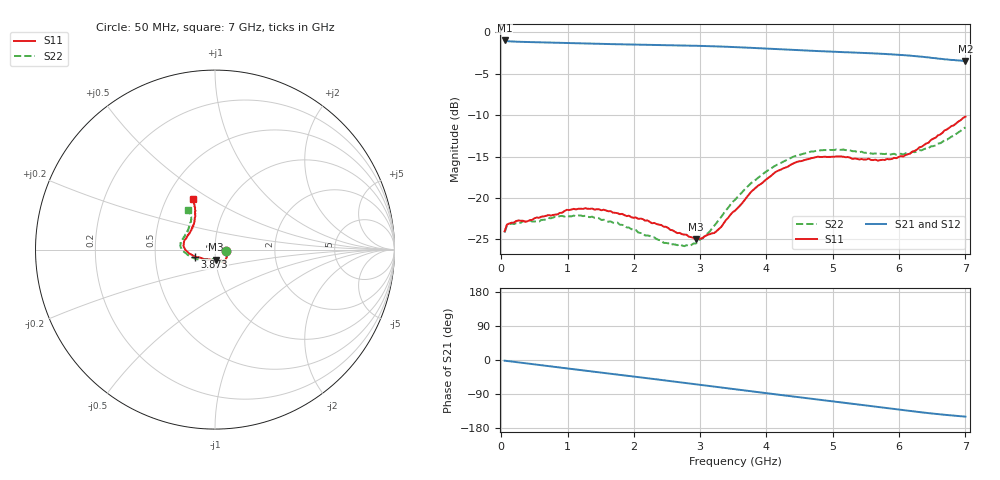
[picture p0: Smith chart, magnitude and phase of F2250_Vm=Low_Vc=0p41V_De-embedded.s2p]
! Integrated Device Technology
! Corporate Headquarters
! 6024 Silver Creek Valley Road
! San Jose, CA 95138  USA
! Phone:  1-408-284-8200
! Toll Free:  1-800-223-1366
! Webpage:  http://www.idt.com/
! Timing and RF Division
! 515 Groton Road, Suite 102
! Westford, MA 01886-6024
! Device:  F2250
! Description: Voltage Variable RF Attenuator
! Frequency:  50.0 -  6000.00 MHz
! Package:  3x3 mm Thin QFN Plastic Package: 16 pin
! Ports:  2 RF, 3 DC
!  Pin  1  = GND
!  Pin  2  = NC
!  Pin  3  = RF1  = Port 1
!  Pin  4  = NC
!  Pin  5  = GND
!  Pin  6  = GND
!  Pin  7  = GND
!  Pin  8  = GND
!  Pin  9  = NC
!  Pin 10  = RF2  = Port 2
!  Pin 11  = NC
!  Pin 12  = GND
!  Pin 13  = GND
!  Pin 14  = VCNTRL
!  Pin 15  = VDD
!  Pin 16  = VMODE
! Vcntrl:  0.410 Volts
! Vmode:  +0.000 Volts
! Vdd:  +3.30  Volts
! Current:  1.125 mA
! Data:  The device was measured on a the F2250 evaluation board which has
!  individual transmission lines to the RF pins.  Data was collected
!  using a calibrated network analyzer.  The evaluation board was
!  de-embedded using a TRL calibration technique.
!  The reference plane is the edge of the package pin.
! Misc:  SN 10
!  Action Tracker AT0258
! Date Measured:  2014-11-26
! Date:  2015-10-15  MJV
! Note:
!  Integrated Device Technology supplies this data as a sample of measured
!  data at the package pin for this product.  Your particular data for this
!  product may vary.
!  Data was taken at 25 degrees C.
!  Integrated Device Technology reserves the right to change this data at anytime.
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# GHz S dB R 50
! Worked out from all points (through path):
!   201 points, 50 MHz to 7 GHz, reference 50 ohm
!   highest |S21| = -1.00 dB at 50 MHz (marker M1); lowest = -3.5 dB at 7 GHz (marker M2)
!   group delay of S21, straight-line fit = 60 ps
!   lowest |S11| = -25.0 dB at 2.934 GHz (marker M3), VSWR 1.12, Z = 50 - j5.63 ohm
!   |S11| at or under -10 dB: start of sweep to end of sweep
!   |S22| runs from -25.8 to -11.5 dB; largest |S21 - S12| = 0.0004
!   S11 on the Smith chart (normalised r, x): 50 MHz: 1.13, -0.02; 3.873 GHz: 0.80, -0.06; 7 GHz: 0.67, +0.42
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0.05  -24.01 -8.7  -1.00 -1.8  -1.00 -1.8  -24.17 -9.3
0.08475  -23.21 -8.6  -1.07 -2.5  -1.07 -2.5  -23.31 -8.7
0.15425  -22.99 -10.8  -1.12 -4.0  -1.12 -4.0  -23.08 -10.4
0.6755  -22.15 -33.5  -1.25 -15.4  -1.24 -15.4  -22.59 -34.9
0.884  -21.80 -42.7  -1.29 -20.0  -1.29 -20.0  -22.18 -45.0
1.2315  -21.32 -52.6  -1.36 -27.4  -1.36 -27.4  -22.19 -57.7
1.75275  -21.82 -59.3  -1.46 -38.4  -1.46 -38.5  -22.97 -65.6
2.37825  -23.23 -60.5  -1.55 -51.8  -1.54 -51.8  -25.07 -69.3
2.552  -23.85 -64.4  -1.57 -55.6  -1.57 -55.6  -25.67 -75.0
2.83  -24.67 -78.2  -1.62 -61.7  -1.62 -61.7  -25.80 -93.1
2.93425  -25.00 -86.3  -1.64 -64.0  -1.64 -64.0  -25.50 -101.3
3.21225  -24.22 -114.9  -1.71 -70.2  -1.70 -70.2  -23.34 -125.9
3.525  -21.53 -142.9  -1.80 -77.1  -1.80 -77.1  -20.22 -144.8
3.8725  -18.52 -160.6  -1.93 -84.8  -1.93 -84.8  -17.56 -160.4
4.1505  -16.80 -170.9  -2.04 -90.9  -2.04 -90.9  -16.02 -170.4
4.4285  -15.76 -178.7  -2.15 -96.9  -2.15 -96.9  -14.95 -177.7
4.7065  -15.15 174.5  -2.25 -102.9  -2.25 -102.9  -14.40 176.2
5.15825  -15.02 163.6  -2.41 -112.6  -2.41 -112.6  -14.16 166.9
5.85325  -15.34 140.3  -2.66 -127.6  -2.66 -127.6  -14.76 151.7
6.166  -14.66 129.1  -2.83 -134.4  -2.83 -134.4  -14.59 142.7
6.444  -13.34 120.5  -3.04 -140.2  -3.04 -140.2  -14.00 133.4
7  -10.19 113.9  -3.48 -149.5  -3.48 -149.5  -11.49 123.9
